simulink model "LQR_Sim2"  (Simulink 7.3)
settings: Solver=ode45  StartTime=0.0  StopTime=100  RelTol=1e-3
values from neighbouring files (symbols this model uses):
  calfa = cosd(alfa)    [LQR_Design.m]
  d2r = pi/180    (= 0.0174532925199)    [LQR_Design.m]    (also in init.m; pl.m)
  ge = 32.174    [LQR_Design.m]
  r2d = 180/pi    (= 57.2957795131)    [LQR_Design.m]    (also in init.m; pl.m)
  salfa = sind(alfa)    [LQR_Design.m]
  Thet0 = 25    [LQR_Design.m]
  V0 = 600    [LQR_Design.m]
undefined symbols (not defined in the file or in its folder): As, Bs, Cs, Ds, Kpr, Kq

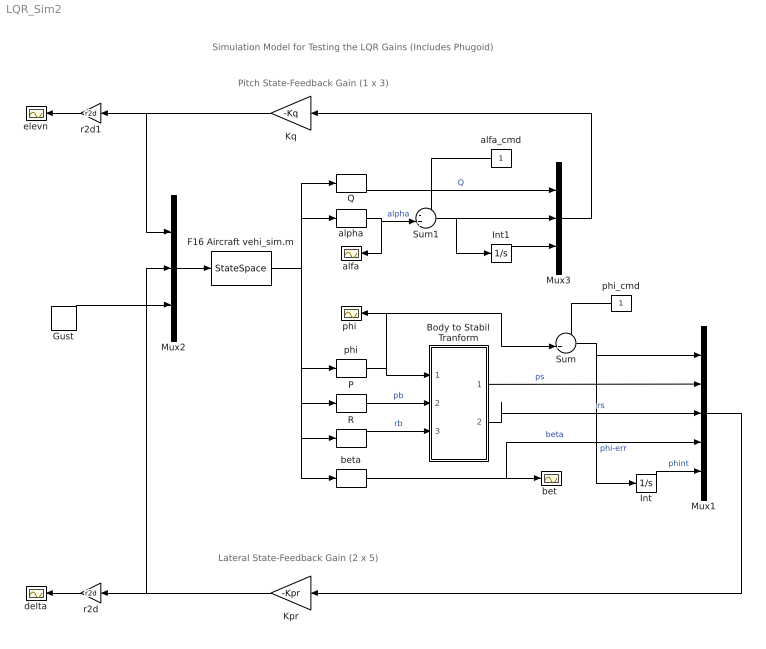
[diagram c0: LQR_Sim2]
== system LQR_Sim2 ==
  note: Simulation Model for Testing the LQR Gains (Includes Phugoid)
  note: Lateral State-Feedback Gain (2 x 5)
  note: Pitch State-Feedback Gain (1 x 3)
  Body to Stabil Tranform : Subsystem
  F16 Aircraft vehi_sim.m : StateSpace  A=As  B=Bs  C=Cs  D=Ds
  Gust : DiscretePulseGenerator  PulseType=Time based  Amplitude=00  Period=500  PulseWidth=2  PhaseDelay=1  SampleTime=1
  Int : Integrator
  Int1 : Integrator
  Kpr : Gain  Gain=-Kpr  Multiplication=Matrix(K*u)  ParameterDataType=fixdt(1, 16)  ParameterScaling=2^0  OutDataType=fixdt(1, 16)  OutScaling=2^0
  Kq : Gain  Gain=-Kq  Multiplication=Matrix(K*u)  ParameterDataType=fixdt(1, 16)  ParameterScaling=2^0  OutDataType=fixdt(1, 16)  OutScaling=2^0
  Mux1 : Mux  Inputs=5
  Mux2 : Mux  Inputs=[1, 2, 1]
  Mux3 : Mux  Inputs=3
  P : Selector  InputPortWidth=14  IndexOptions=Index vector (dialog)  Indices=[2]  OutputSizes=1
  Q : Selector  InputPortWidth=14  IndexOptions=Index vector (dialog)  Indices=[4]  OutputSizes=1
  R : Selector  InputPortWidth=14  IndexOptions=Index vector (dialog)  Indices=[6]  OutputSizes=1
  Sum : Sum  Inputs=-+|  OutDataType=fixdt(1, 16)  OutScaling=2^0
  Sum1 : Sum  Inputs=-+|  OutDataType=fixdt(1, 16)  OutScaling=2^0
  alfa : Scope
  alfa_cmd : Constant  OutDataType=fixdt(1, 16)  OutScaling=2^0
  alpha : Selector  InputPortWidth=14  IndexOptions=Index vector (dialog)  Indices=[7]  OutputSizes=1
  "bet " : Scope
  beta : Selector  InputPortWidth=14  IndexOptions=Index vector (dialog)  Indices=[8]  OutputSizes=1
  delta : Scope
  elevn : Scope
  phi : Selector  InputPortWidth=14  IndexOptions=Index vector (dialog)  Indices=[1]  OutputSizes=1
  "phi " : Scope
  phi_cmd : Constant  OutDataType=fixdt(1, 16)  OutScaling=2^0
  r2d : Gain  Gain=r2d  ParameterDataType=fixdt(1, 16)  ParameterScaling=2^0  OutDataType=fixdt(1, 16)  OutScaling=2^0
  r2d1 : Gain  Gain=r2d  ParameterDataType=fixdt(1, 16)  ParameterScaling=2^0  OutDataType=fixdt(1, 16)  OutScaling=2^0
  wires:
  Sum/1 -> Mux1/1, Int/1  "phi-err"
  phi_cmd/1 -> Sum/1
  Mux1/1 -> Kpr/1
  r2d/1 -> delta/1
  Mux2/1 -> F16 Aircraft vehi_sim.m/1
  F16 Aircraft vehi_sim.m/1 -> alpha/1, Q/1, phi/1, P/1, R/1, beta/1
  Mux3/1 -> Kq/1
  phi/1 -> "phi "/1, Sum/2, Body to Stabil Tranform/1(phi)
  Kpr/1 -> Mux2/2, r2d/1
  r2d1/1 -> elevn/1
  Int1/1 -> Mux3/3
  Q/1 -> Mux3/1  "Q"
  Sum1/1 -> Mux3/2, Int1/1
  alpha/1 -> Sum1/2, alfa/1  "alpha"
  Kq/1 -> r2d1/1, Mux2/1
  beta/1 -> Mux1/4, "bet "/1  "beta"
  alfa_cmd/1 -> Sum1/1
  Gust/1 -> Mux2/3
  P/1 -> Body to Stabil Tranform/2(p_b)  "pb"
  R/1 -> Body to Stabil Tranform/3(r_b)  "rb"
  Body to Stabil Tranform/1(p_s) -> Mux1/2  "ps"
  Body to Stabil Tranform/2(r_s) -> Mux1/3  "rs"
  Int/1 -> Mux1/5  "phint"

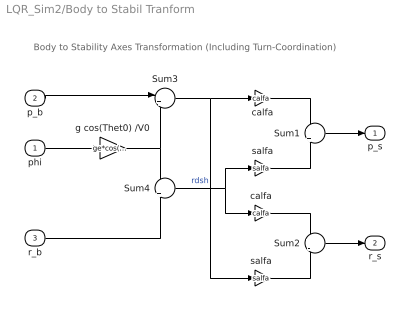
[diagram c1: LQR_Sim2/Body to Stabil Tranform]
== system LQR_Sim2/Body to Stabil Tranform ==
  note: Body to Stability Axes Transformation (Including Turn-Coordination)
  phi : Inport  OutDataType=sfix(16)  OutScaling=2^0
  p_b : Inport  Port=2  OutDataType=sfix(16)  OutScaling=2^0
  r_b : Inport  Port=3  OutDataType=sfix(16)  OutScaling=2^0
  Sum1 : Sum  Inputs=+|+  OutDataType=sfix(16)  OutScaling=2^0
  Sum2 : Sum  Inputs=+|-  OutDataType=sfix(16)  OutScaling=2^0
  Sum3 : Sum  Inputs=|++  OutDataType=sfix(16)  OutScaling=2^0
  Sum4 : Sum  Inputs=-|+  OutDataType=sfix(16)  OutScaling=2^0
  calfa : Gain  Gain=calfa  ParameterDataType=sfix(16)  ParameterScaling=2^0  OutDataType=sfix(16)  OutScaling=2^0
  "calfa " : Gain  Gain=calfa  ParameterDataType=sfix(16)  ParameterScaling=2^0  OutDataType=sfix(16)  OutScaling=2^0
  g cos(Thet0) /V0 : Gain  Gain=ge*cos(Thet0*d2r)/V0  ParameterDataType=sfix(16)  ParameterScaling=2^0  OutDataType=sfix(16)  OutScaling=2^0
  salfa : Gain  Gain=salfa  ParameterDataType=sfix(16)  ParameterScaling=2^0  OutDataType=sfix(16)  OutScaling=2^0
  "salfa " : Gain  Gain=salfa  ParameterDataType=sfix(16)  ParameterScaling=2^0  OutDataType=sfix(16)  OutScaling=2^0
  p_s : Outport  OutDataType=sfix(16)  OutScaling=2^0
  r_s : Outport  Port=2  OutDataType=sfix(16)  OutScaling=2^0
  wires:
  "salfa "/1 -> Sum2/2
  "calfa "/1 -> Sum2/1
  salfa/1 -> Sum1/2
  calfa/1 -> Sum1/1
  Sum3/1 -> calfa/1, "salfa "/1
  Sum4/1 -> salfa/1, "calfa "/1  "rdsh"
  p_b/1 -> Sum3/1
  Sum1/1 -> p_s/1
  Sum2/1 -> r_s/1
  r_b/1 -> Sum4/2
  g cos(Thet0) /V0/1 -> Sum4/1, Sum3/2
  phi/1 -> g cos(Thet0) /V0/1
